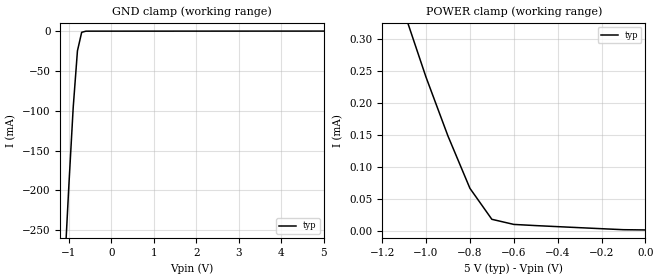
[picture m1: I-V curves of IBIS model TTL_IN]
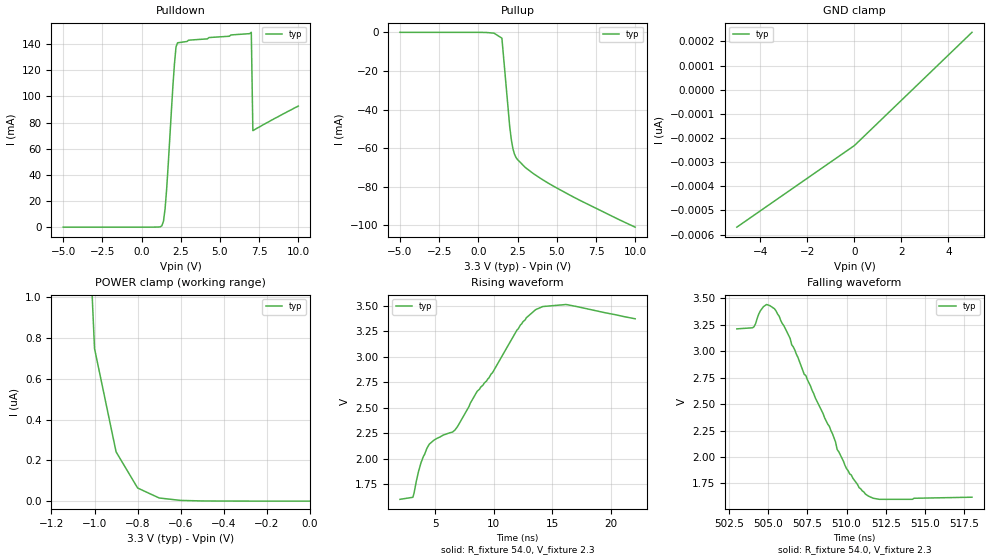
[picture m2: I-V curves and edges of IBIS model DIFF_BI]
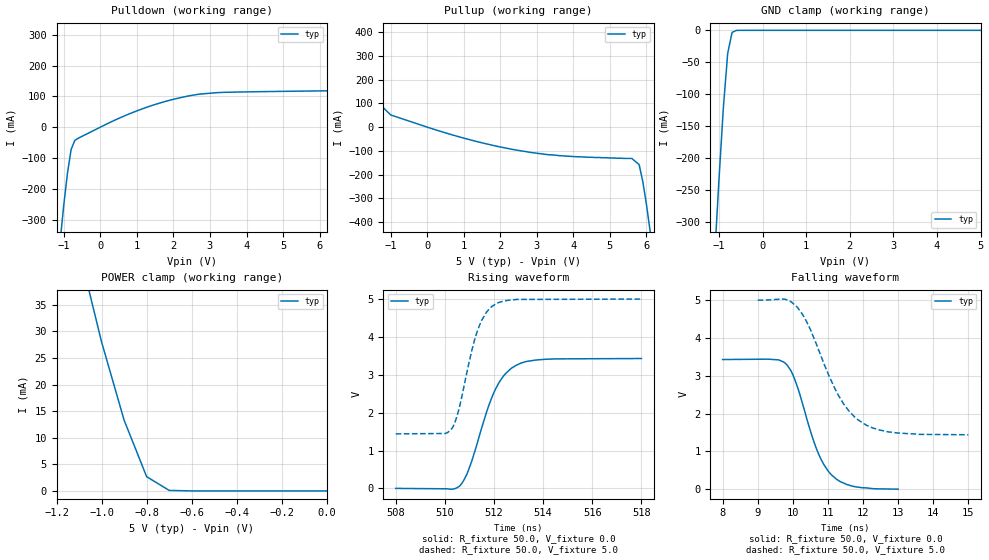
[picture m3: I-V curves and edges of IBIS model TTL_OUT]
|   Texas Instruments Incorporated
|   Data Transmissions Products
|   IBIS Model for SN75LBC171
|   20pin SOIC Package
[IBIS Ver]   3.2
[Comment char]   |_char
[File name]   lbc171dw.ibs
[File Rev]   2.0
[Date]   18Jan01
[Source]   File originated at Texas Instruments Incorporated.
   Data Transmission Products Group. All data based on
   Bench Measurements.
[Notes]
[Disclaimer]
(C) Copyright Texas Instruments Incorporated 2001
   All rights reserved
  Texas Instruments Incorporated hereby grants the user of this IBIS
model a non-exclusive, nontransferable license to use this IBIS model
under the following terms.  Before using this IBIS model, the user
should read this license.  If the user does not accept these terms,
the IBIS model should be returned to Texas Instruments within 30 days.
  The user is granted this license only to use the IBIS model and
is not granted rights to sell, load, rent, lease or license the IBIS
model in whole or in part, or in modified form to anyone other than
user.  User may modify the IBIS model to suit its specific applications
but rights to derivative works and such modifications shall belong to
Texas Instruments.
  This IBIS model is provided on an "AS IS" basis and Texas Instruments
makes absolutely no warranty with respect to the information contained
herein.  TEXAS INSTRUMENTS DISCLAIMS AND CUSTOMER WAIVES ALL WARRANTIES,
EXPRESS OR IMPLIED, INCLUDING WARRANTIES OF MERCHANTABILITY OR FITNESS
FOR A PARTICULAR PURPOSE. The entire risk as to quality and performance
is with the Customer. ACCORDINGLY, IN NO EVENT SHALL THE COMPANY BE LIABLE
FOR ANY DAMAGES, WHETHER IN CONTRACT OR TORT,INCLUDING ANY LOST PROFITS
OR OTHER INCIDENTAL, CONSEQUENTIAL, EXEMPLARY, OR PUNITIVE DAMAGES ARISING
OUT OF THE USE OR APPLICATION OF THE IBIS model provided in this package.
Further, Texas Instruments reserves the right to discontinue or make changes
without notice to any product herein to improve reliability, function, or
design. Texas Instruments does not convey any license under patent rights
or any other intellectual property rights, including those of third parties.
Contact Texas Instruments at ATTN:DATA TRANSMISSIONS
[Copyright]   Copyright 2001, Texas Instruments, All Rights Reserved
[Component]   SN75LBC171DW
[Manufacturer]  Texas Instruments Incorporated
[Package]
|   typ   min   max
R_pkg   0.038   0.033   0.045
L_pkg   5.012nH   4.110nH   6.349nH
C_pkg   0.717pF   0.530pF   0.868pF
[Pin]   signal_name   model_name   R_pin   L_pin   C_pin
1   1R   TTL_OUT   0.042   6.336n   0.865p
2   1DE   TTL_IN   0.043   5.542n   0.867p
3   1D   TTL_IN   0.034   4.714n   0.732p
4   GND   GND   0.034   4.377n   0.591p
5   GND   GND   0.036   4.130n   0.533p
6   2R   TTL_OUT   0.035   4.111n   0.530p
7   2DE   TTL_IN   0.034   4.284n   0.583p
8   2D   TTL_IN   0.034   4.634n   0.726p
9   3R   TTL_OUT   0.040   5.518n   0.865p
10   3DE   TTL_IN   0.043   6.349n   0.866p
11   3D   TTL_IN   0.041   6.281n   0.861p
12   3A   DIFF_BI   0.045   5.561n   0.868p
13   3B   DIFF_BI   0.033   4.778n   0.742p
14   2A   DIFF_BI   0.035   4.414n   0.596p
15   2B   DIFF_BI   0.035   4.110n   0.533p
16   VCC   POWER   0.036   4.130n   0.533p
17   CDE   TTL_IN   0.034   4.377n   0.591p
18   /RE   TTL_IN   0.034   4.714n   0.731p
19   1A   DIFF_BI   0.043   5.569n   0.868p
20   1B   DIFF_BI   0.042   6.308n   0.864p
[Diff_pin]   inv_pin   vdiff   tdelay_typ   tdelay_min   tdelay_max
| The 'xA' pin is Diff_pin and the 'xB' pin is the inv_pin
12   13   100mV   0 0 0
14   15   100mV   0 0 0
19   20   100mV   0 0 0
| Models and submodels in the file (3): TTL_IN (Input), DIFF_BI (I/O), TTL_OUT (3-state)
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|   TTL Input Model
[Model]   TTL_IN
Model_type   Input
|Signals   CDE,1DE,1D,/RE,2DE,2D,3DE,3D
Vinh = 2.0
Vinl = 0.8
|   typ   min   max
C_comp   1.0pF   NA   NA
|   typ   min   max
[Temperature Range]   25.0   NA   NA
[Voltage range]   5.0V   4.75V   5.25V
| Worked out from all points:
|   GND clamp passes 1 mA (typ) near -0.67 V on its own axis
[GND_clamp]
|   Voltage   I(typ)   I(min)   I(max)
-5V       -4.21A     NA         NA
-2V       -1.22A     NA         NA
-1V       -192mA     NA         NA
-900mV    -96.1mA    NA         NA
-800mV    -24.8mA    NA         NA
-700mV    -1.47mA    NA         NA
-500mV    -28.2uA    NA         NA
5V        57.8uA     NA         NA
[Power_clamp]
| Note that the[POWER_clamp]voltage table is referenced to Vcc
| and is calculated using Vtable=Vcc - Vmeasured.
|   Voltage   I(typ)   I(min)   I(max)
-5V       4.42mA     NA         NA
-2V       1.26mA     NA         NA
-1V       240uA      NA         NA
-900mV    148uA      NA         NA
-800mV    66.3uA     NA         NA
-700mV    17.8uA     NA         NA
-600mV    9.8uA      NA         NA
-100mV    1.53uA     NA         NA
0V        1.16uA     NA         NA
|   Driver Output/Receiver Input Model
[Model]   DIFF_BI
Model_type   I/O
| Signals   1A,1B,2A,2B,3A,3B
Vinl = 1.0V
Vinh = 1.4V
Vmeas = 2.3V   |Reference voltage for timing measurements
Cref = 50pF   |Timing specification test load capacitance value
Rref = 54   |Note: 54 Ohm load; single ended configuration
| variable   typ   min   max
C_comp   1.0pF   NA   NA
|   typ   min   max
[Temperature Range]   25.0   NA   NA
[Voltage range]   3.3V   3.0V   3.6V
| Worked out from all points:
|   slope of the pulldown table from 0 to 0.495 V, typ, clamps not added: 57.6 kohm
|   slope of the pullup table from 0 to 0.495 V, typ, clamps not added: 8.29 kohm
|   rising waveform, R_fixture 54.0, V_fixture 2.3: 20-80 % time 7ns typ, NA min, NA max; typ from 1.6 V to 3.37 V
|   falling waveform, R_fixture 54.0, V_fixture 2.3: 20-80 % time 2.84ns typ, NA min, NA max; typ from 3.21 V to 1.62 V
[Pulldown]
|   Voltage   I(typ)   I(min)   I(max)
-5V       -560pA     NA         NA
1.3V      1.13mA     NA         NA
1.4V      4.65mA     NA         NA
1.5V      13.9mA     NA         NA
1.6V      29mA       NA         NA
2V        108mA      NA         NA
2.1V      125mA      NA         NA
2.2V      138mA      NA         NA
2.3V      141mA      NA         NA
7V        149mA      NA         NA
7.1V      73.8mA     NA         NA
10V       92.6mA     NA         NA
[Pullup]
|   Voltage   I(typ)   I(min)   I(max)
| Note that the[Pullup]voltage table is referenced to Vcc
| and is calculated using Vtable=Vcc - Vmeasured.
-5V       16.6uA     NA         NA
500mV     -60.3uA    NA         NA
1V        -426uA     NA         NA
1.5V      -3.01mA    NA         NA
2V        -49mA      NA         NA
2.1V      -55.5mA    NA         NA
2.2V      -60.2mA    NA         NA
2.4V      -64.9mA    NA         NA
3V        -70.1mA    NA         NA
4.5V      -78.4mA    NA         NA
6.5V      -87.2mA    NA         NA
10V       -101mA     NA         NA
| Output in High Impedance (off)
[GND_clamp]
|   Voltage   I(typ)   I(min)   I(max)
-5V       -569pA     NA         NA
0V        -231pA     NA         NA
5V        238pA      NA         NA
[POWER_clamp]
|   Voltage   I(typ)   I(min)   I(max)
| Note that the [POWER_clamp] voltage table is referenced to Vcc
| and is calculated using Vtable = Vcc - Vmeasured.
| Outputs in Tri-state.
-5V       16.6uA     NA         NA
-1.5V     12.7uA     NA         NA
-1V       749nA      NA         NA
-900mV    242nA      NA         NA
-800mV    64.6nA     NA         NA
-700mV    15.6nA     NA         NA
-600mV    3.78nA     NA         NA
0V        238pA      NA         NA
[Ramp]
|   typ   min   max
dV/dt_r   1.77v/7ns   NA   NA
dV/dt_f   1.60v/3.2ns   NA   NA
R_load = 54ohm  | Note: The measurement is single-ended with respect
|   to ground.
[Rising Waveform]
R_fixture = 54.0
V_fixture = 2.3
C_fixture = 0p
L_fixture = 0n
|   V(typ)   V(min)   V(max)
2ns       1.6V       NA         NA
3.1ns     1.62V      NA         NA
3.8ns     1.96V      NA         NA
4.5ns     2.14V      NA         NA
6.7ns     2.28V      NA         NA
9.9ns     2.84V      NA         NA
12ns      3.26V      NA         NA
13.6ns    3.46V      NA         NA
16.2ns    3.51V      NA         NA
22.1ns    3.37V      NA         NA
[Falling Waveform]
R_fixture = 54.0
V_fixture = 2.3
C_fixture = 0p
L_fixture = 0n
|   V(typ)   V(min)   V(max)
503ns     3.21V      NA         NA
504.1ns   3.23V      NA         NA
504.5ns   3.38V      NA         NA
504.9ns   3.44V      NA         NA
505.4ns   3.4V       NA         NA
508.9ns   2.29V      NA         NA
509.4ns   2.07V      NA         NA
511.2ns   1.65V      NA         NA
512.1ns   1.6V       NA         NA
518ns     1.62V      NA         NA
|   Receiver Output Model
[Model]   TTL_OUT
Model_type   3-state
| Signals   1R,2R,3R
Vmeas = 1.5V   |Reference voltage for timing measurements
Cref = 15pF   |Timing specification test load capacitance value
Vref = 0   |Timing specification test load voltage; GND
| variable   typ   min   max
C_comp   1.0pF   NA   NA
|   typ   min   max
[Temperature Range]   25.0   NA   NA
[Voltage range]   5.0V   4.75V   5.25V
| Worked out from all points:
|   slope of the pulldown table from 0 to 0.75 V, typ, clamps not added: 18.3 ohm
|   slope of the pullup table from 0 to 0.75 V, typ, clamps not added: 21.1 ohm
|   GND clamp passes 1 mA (typ) near -0.63 V on its own axis
|   POWER clamp passes 1 mA (typ) near -0.73 V on its own axis
|   rising waveform, R_fixture 50.0, V_fixture 0.0: 20-80 % time 1.09ns typ, NA min, NA max; typ from 0 V to 3.43 V
|   falling waveform, R_fixture 50.0, V_fixture 0.0: 20-80 % time 747ps typ, NA min, NA max; typ from 3.43 V to 0 V
|   rising waveform, R_fixture 50.0, V_fixture 5.0: 20-80 % time 802ps typ, NA min, NA max; typ from 1.44 V to 5 V
|   falling waveform, R_fixture 50.0, V_fixture 5.0: 20-80 % time 1.06ns typ, NA min, NA max; typ from 5 V to 1.44 V
[Pulldown]
|   Voltage   I(typ)   I(min)   I(max)
-5V       -4.96A     NA         NA
-2V       -1.44A     NA         NA
-1V       -251mA     NA         NA
-900mV    -149mA     NA         NA
-800mV    -72.1mA    NA         NA
-700mV    -43mA      NA         NA
400mV     22.9mA     NA         NA
2.7V      107mA      NA         NA
6.3V      118mA      NA         NA
6.6V      139mA      NA         NA
7.7V      328mA      NA         NA
10V       741mA      NA         NA
[Pullup]
|   Voltage   I(typ)   I(min)   I(max)
| Note that the[Pullup]voltage table is referenced to Vcc
| and is calculated using Vtable=Vcc - Vmeasured.
-5V       740mA      NA         NA
-4V       560mA      NA         NA
-3V       380mA      NA         NA
-2V       202mA      NA         NA
-1V       51.4mA     NA         NA
2.4V      -95.6mA    NA         NA
5.6V      -132mA     NA         NA
5.8V      -158mA     NA         NA
5.9V      -229mA     NA         NA
6V        -326mA     NA         NA
7V        -1.44A     NA         NA
10V       -4.96A     NA         NA
| Output in High Impedance (off)
[GND_clamp]
|   Voltage   I(typ)   I(min)   I(max)
-5V       -4.96A     NA         NA
-2V       -1.44A     NA         NA
-1V       -233mA     NA         NA
-900mV    -121mA     NA         NA
-800mV    -35.7mA    NA         NA
-700mV    -3.28mA    NA         NA
-600mV    -151uA     NA         NA
5V        66.5pA     NA         NA
[POWER_clamp]
|   Voltage   I(typ)   I(min)   I(max)
| Note that the [POWER_clamp] voltage table is referenced to Vcc
| and is calculated using Vtable = Vcc - Vmeasured.
| Outputs in Tri-state.
-5V       740mA      NA         NA
-2V       201mA      NA         NA
-1V       28mA       NA         NA
-900mV    13.3mA     NA         NA
-800mV    2.68mA     NA         NA
-700mV    98.5uA     NA         NA
0V        66.5pA     NA         NA
[Ramp]
|   typ   min   max
dV/dt_r   2.54v/1.2ns   NA   NA
dV/dt_f   2.14v/1.0ns   NA   NA
R_load = 50Ohm
[Rising Waveform]
R_fixture = 50.0
V_fixture = 0.0
C_fixture = 0p
L_fixture = 0n
|   V(typ)   V(min)   V(max)
508ns     0V         NA         NA
510.3ns   -20mV      NA         NA
510.6ns   60mV       NA         NA
511ns     550mV      NA         NA
511.7ns   2.02V      NA         NA
512ns     2.54V      NA         NA
512.4ns   2.98V      NA         NA
512.9ns   3.25V      NA         NA
514.1ns   3.41V      NA         NA
518ns     3.43V      NA         NA
[Falling Waveform]
R_fixture = 50.0
V_fixture = 0.0
C_fixture = 0p
L_fixture = 0n
|   V(typ)   V(min)   V(max)
8ns       3.43V      NA         NA
9.3ns     3.44V      NA         NA
9.75ns    3.36V      NA         NA
9.95ns    3.13V      NA         NA
10.05ns   2.92V      NA         NA
10.65ns   1.13V      NA         NA
10.85ns   710mV      NA         NA
11.05ns   430mV      NA         NA
11.65ns   90mV       NA         NA
13ns      0V         NA         NA
[Rising Waveform]
R_fixture = 50.0
V_fixture = 5.0
C_fixture = 0p
L_fixture = 0n
|   V(typ)   V(min)   V(max)
508ns     1.44V      NA         NA
510ns     1.45V      NA         NA
510.3ns   1.59V      NA         NA
510.6ns   2.16V      NA         NA
511.1ns   3.65V      NA         NA
511.3ns   4.11V      NA         NA
511.7ns   4.66V      NA         NA
512.1ns   4.89V      NA         NA
512.9ns   4.99V      NA         NA
518ns     5V         NA         NA
[Falling Waveform]
R_fixture = 50.0
V_fixture = 5.0
C_fixture = 0p
L_fixture = 0n
|   V(typ)   V(min)   V(max)
9ns       5V         NA         NA
9.75ns    5.03V      NA         NA
10.15ns   4.79V      NA         NA
10.5ns    4.23V      NA         NA
11.05ns   2.96V      NA         NA
11.3ns    2.48V      NA         NA
11.6ns    2.07V      NA         NA
12ns      1.74V      NA         NA
12.75ns   1.51V      NA         NA
15ns      1.44V      NA         NA
